(* 	
	Program Name: 	ACS_MOVE_INCREMENTAL_LINEAR_POSITIVE
	Purpose:		Copy Incremental Move Profile to ACS Drive Output Registers
	When Executed:	Primes Output Registers for an Incremental Move in the Positive Direction to be executed upon Start Motion command
*)
PROGRAM ACS_MOVE_INCREMENTAL_LINEAR_POSITIVE
VAR_IN_OUT
	Axis:ACS_DRIVE_TYPE;
END_VAR

VAR_INPUT
	// Distance to move in mm or rotary units
	ProfileDistance		:REAL;
	// Velocity in mm/s or rotary units
	ProfileVelocity		:REAL;
	// Acceleration in mm/s*s or rotary units
	ProfileAcceleration	:REAL;
	//Deceleration in mm/s*s or rotary units
	ProfileDeceleration	:REAL;
	// Force as % Peak motor current
	ProfileForce		:REAL;
END_VAR

VAR
	_moveType:UDINT := ACS_MOTION_TYPES.INCREMENTAL_POSITIVE;
	// Target Index
	_moveSelect:USINT := 0;
END_VAR

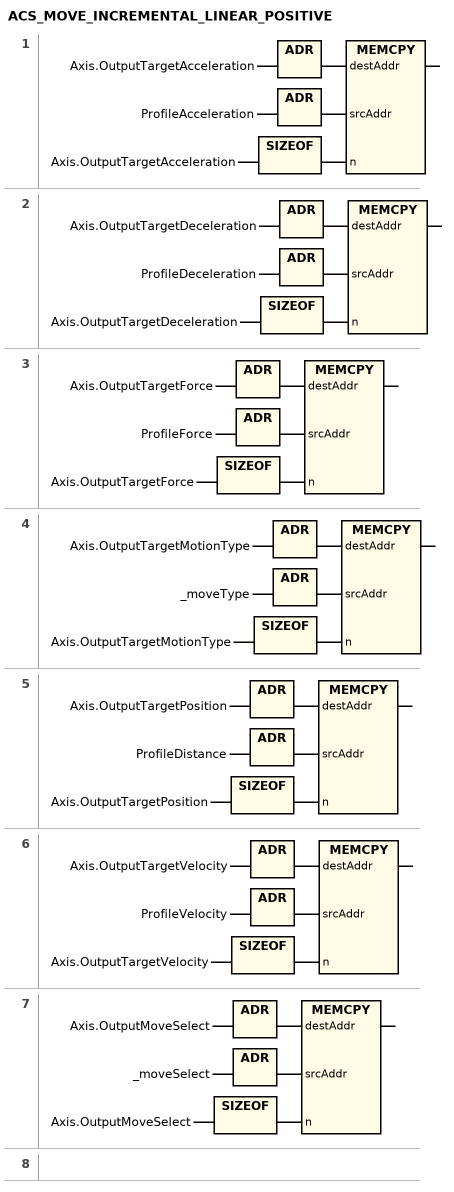
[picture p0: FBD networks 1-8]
// NETWORK 1
MEMCPY(destAddr := ADR(Axis.OutputTargetAcceleration), srcAddr := ADR(ProfileAcceleration), n := SIZEOF(Axis.OutputTargetAcceleration));

// NETWORK 2
MEMCPY(destAddr := ADR(Axis.OutputTargetDeceleration), srcAddr := ADR(ProfileDeceleration), n := SIZEOF(Axis.OutputTargetDeceleration));

// NETWORK 3
MEMCPY(destAddr := ADR(Axis.OutputTargetForce), srcAddr := ADR(ProfileForce), n := SIZEOF(Axis.OutputTargetForce));

// NETWORK 4
MEMCPY(destAddr := ADR(Axis.OutputTargetMotionType), srcAddr := ADR(_moveType), n := SIZEOF(Axis.OutputTargetMotionType));

// NETWORK 5
MEMCPY(destAddr := ADR(Axis.OutputTargetPosition), srcAddr := ADR(ProfileDistance), n := SIZEOF(Axis.OutputTargetPosition));

// NETWORK 6
MEMCPY(destAddr := ADR(Axis.OutputTargetVelocity), srcAddr := ADR(ProfileVelocity), n := SIZEOF(Axis.OutputTargetVelocity));

// NETWORK 7
MEMCPY(destAddr := ADR(Axis.OutputMoveSelect), srcAddr := ADR(_moveSelect), n := SIZEOF(Axis.OutputMoveSelect));

// NETWORK 8

END_PROGRAM
